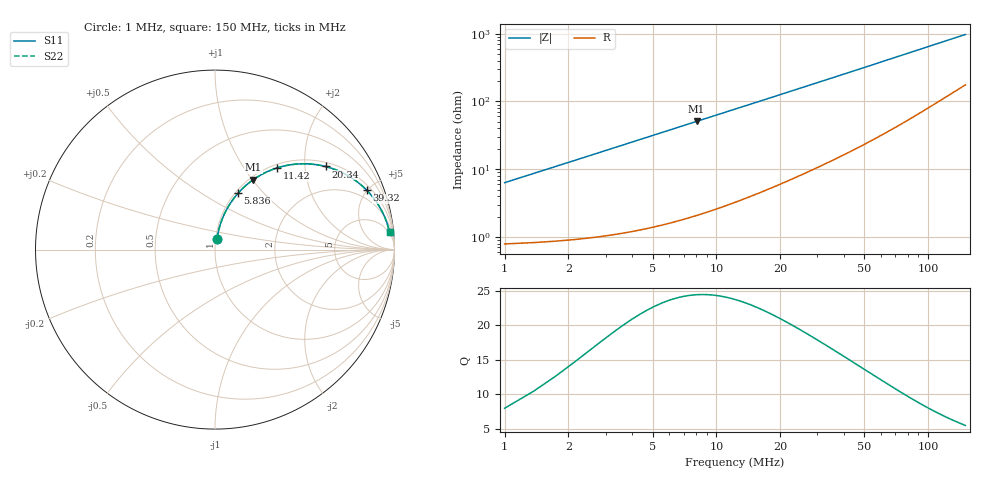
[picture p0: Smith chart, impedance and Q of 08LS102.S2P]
! Coilcraft 0805LS-102 Chip Inductor
! 18 September 2002
# MHZ S MA R 50
!Freq  MagS11  AngS11  MagS21  AngS21  MagS12  AngS12  MagS22  AngS22
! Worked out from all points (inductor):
!   402 points, 1 MHz to 150 MHz, reference 50 ohm
!   read as one part in series: L = 1 uH near 1.744 MHz
!   highest Q = 24.4 at 8.068 MHz (marker M1), where L = 1 uH
!   S11 on the Smith chart (normalised r, x): 1 MHz: 1.02, +0.13; 5.836 MHz: 1.03, +0.73; 11.42 MHz: 1.06, +1.43; 20.34 MHz: 1.12, +2.56; 39.32 MHz: 1.32, +4.96; 150 MHz: 5, +19
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1  0.0627 79.3  0.9902 -3.6  0.9902 -3.6  0.0627 79.3
1.372  0.08557 79.6  0.9882 -4.9  0.9882 -4.9  0.08557 79.6
2.116  0.1309 78.6  0.9825 -7.5  0.9825 -7.5  0.1309 78.6
2.488  0.1533 77.7  0.9788 -8.8  0.9788 -8.8  0.1533 77.7
3.232  0.1972 75.6  0.97 -11.4  0.97 -11.4  0.1972 75.6
4.348  0.2607 72.3  0.9534 -15.1  0.9534 -15.1  0.2607 72.3
5.836  0.3398 67.7  0.9262 -19.8  0.9262 -19.8  0.3398 67.7
6.952  0.3945 64.4  0.9027 -23.2  0.9027 -23.2  0.3945 64.4
8.068  0.445 61.3  0.8775 -26.4  0.8775 -26.4  0.445 61.3
9.556  0.5059 57.3  0.8421 -30.4  0.8421 -30.4  0.5059 57.3
11.416  0.5719 52.8  0.7968 -34.8  0.7968 -34.8  0.5719 52.8
15.136  0.6748 45.1  0.7089 -42.4  0.7089 -42.4  0.6748 45.1
20.344  0.7704 36.9  0.6017 -50.3  0.6017 -50.3  0.7704 36.9
25.924  0.8336 30.6  0.5104 -56.3  0.5104 -56.3  0.8336 30.6
31.876  0.8756 25.8  0.4354 -60.9  0.4354 -60.9  0.8756 25.8
39.316  0.9079 21.4  0.3653 -65.0  0.3653 -65.0  0.9079 21.4
50.848  0.9358 16.8  0.29 -68.9  0.29 -68.9  0.9358 16.8
62.752  0.9512 13.7  0.2379 -71.4  0.2379 -71.4  0.9512 13.7
75.772  0.9609 11.4  0.1982 -73.0  0.1982 -73.0  0.9609 11.4
100.696  0.9703 8.5  0.1495 -74.3  0.1495 -74.3  0.9703 8.5
125.248  0.9746 6.8  0.1202 -74.4  0.1202 -74.4  0.9746 6.8
150  0.977 5.7  0.1004 -73.9  0.1004 -73.9  0.977 5.7
